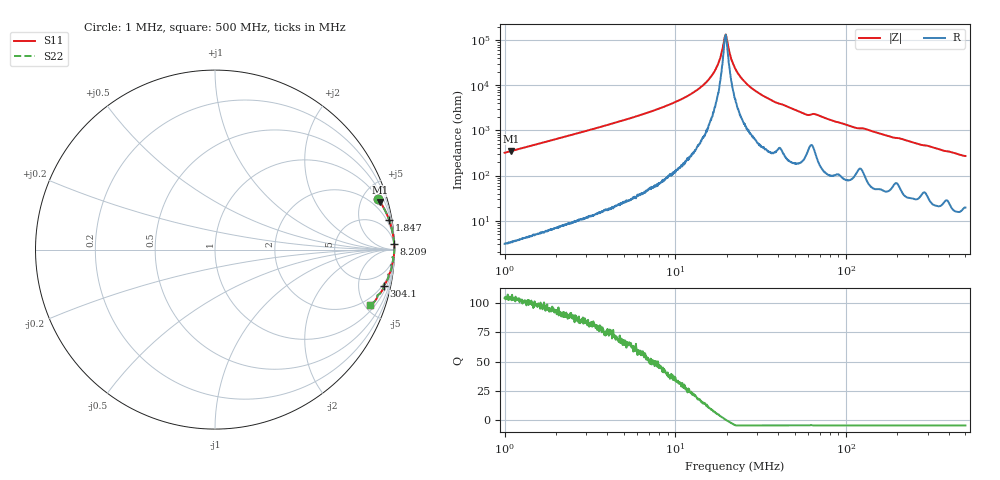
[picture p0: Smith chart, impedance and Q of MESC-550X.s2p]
!s-Parameter Generated by FASTRON Sdn. Bhd.
!FASTRON P/N : MESC-550X
!Keysight Technologies,E4991B,MY54100416,A.01.15
!Date: Fri Mar 27 09:39:09 2026
!Version  : Rev00 Fri Mar 27 09:39:09 2026
!Data & Calibration Information:
!PortZ  Port1:50+j0  Port2:50+j0
!When reading, reference impedance value at option line is always used.
! Remarks : This data is being provided solely for informational purposes.
!Freq	S11	S21	S12	S22
# Hz S dB R 50
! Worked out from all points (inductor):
!   1601 points, 1 MHz to 500 MHz, reference 50 ohm
!   read as one part in series: L = 50.8 uH near 1.032 MHz
!   highest Q = 105 at 1.089 MHz (marker M1), where L = 51 uH
!   self-resonance near 19.67 MHz
!   S11 on the Smith chart (normalised r, x): 1 MHz: 1.06, +6.41; 1.847 MHz: 1, +12; 8.209 MHz: 2, +63; 304.1 MHz: 1.62, -9.01; 500 MHz: 1.39, -5.42
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1000000  -0.43 17.3  -10.54 -72.2  -10.54 -72.2  -0.43 17.3
1089208  -0.36 15.9  -11.23 -73.5  -11.23 -73.5  -0.36 15.9
1847240  -0.14 9.5  -15.62 -79.9  -15.62 -79.9  -0.14 9.5
2820919  -0.06 6.2  -19.30 -83.1  -19.30 -83.1  -0.06 6.2
7957584  -0.01 1.9  -29.60 -86.8  -29.60 -86.8  -0.01 1.9
8208732  -0.01 1.8  -29.97 -86.9  -29.97 -86.9  -0.01 1.8
1.19183e7  -0.01 1.0  -35.50 -86.9  -35.50 -86.9  -0.01 1.0
1.522251e7  -0.01 0.5  -41.49 -84.6  -41.49 -84.6  -0.01 0.5
1.757519e7  -0.01 0.2  -48.53 -78.2  -48.53 -78.2  -0.01 0.2
1.834237e7  -0.01 0.1  -52.16 -71.7  -52.16 -71.7  -0.01 0.1
1.929232e7  -0.01 0.0  -59.83 -38.2  -59.83 -38.2  -0.01 0.0
1.967065e7  -0.01 0.0  -62.10 -2.3  -62.10 -2.3  -0.01 0.0
2.00564e7  -0.01 -0.0  -60.26 36.9  -60.26 36.9  -0.01 -0.0
2.125964e7  -0.01 -0.1  -51.67 71.5  -51.67 71.5  -0.01 -0.1
2.236068e7  -0.01 -0.2  -47.62 77.8  -47.62 77.8  -0.01 -0.2
2.57165e7  -0.01 -0.5  -41.25 83.2  -41.25 83.2  -0.01 -0.5
3.184116e7  -0.01 -0.9  -35.92 85.1  -35.92 85.1  -0.01 -0.9
5.72406e7  -0.05 -2.4  -27.39 81.6  -27.39 81.6  -0.05 -2.4
6.307767e7  -0.09 -2.4  -27.30 75.7  -27.30 75.7  -0.09 -2.4
1.77937e8  -0.15 -7.6  -17.57 78.9  -17.57 78.9  -0.15 -7.6
3.041252e8  -0.33 -12.3  -13.42 73.8  -13.42 73.8  -0.33 -12.3
5e8  -0.75 -19.7  -9.43 66.2  -9.43 66.2  -0.75 -19.7
